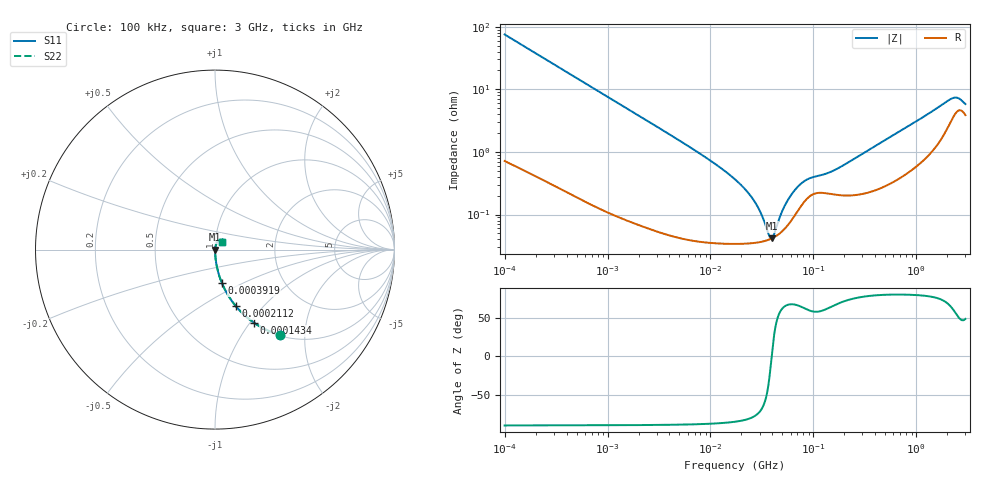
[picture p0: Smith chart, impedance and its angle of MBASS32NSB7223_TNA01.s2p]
! MBASS32NSB7223_TNA01  S-PARAMETER MODEL  ( Standard Model )
! Model Generated by TAIYO YUDEN Corporation (http://www.ty-top.com)
! Version 1.0
! TAIYO YUDEN Control No. 220601
! Copyright(c) 2013 TAIYO YUDEN CO.,LTD. All Rights Reserved.
! Product Description (link to TY-COMPAS)
! https://ds.yuden.co.jp/TYCOMPAS/or/detail?pn=MBASS32NSB7223KTNA01&u=M
! Products Name : Multilayer Ceramic Capacitors
! Characteristics :
!  Capacitance : 0.022 [uF] , Rated Voltage : 630 [V] , TCC : X7R
!  Case Size : 3.2 x 2.5 / 0.126 x 0.098 [mm/inch] , Thickness : 1.9 / 0.075 [mm/inch]
!  (Conditions: Temperature = 25 [degC] , DC Bias Voltage = 0 [V])
! External Node Assignments :
!  1  o---| |---o  2
! GND o---------o GND
! Frequency Range : 100kHz  -  3GHz  [ 401 STEP ]
# MHZ S RI R 50
! Freq[MHz].  S11 Real  S11 Imag  S21 Real  S21 Imag  S12 Real  S12 Imag  S22 Real  S22 Imag
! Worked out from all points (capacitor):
!   401 points, 100 kHz to 3 GHz, reference 50 ohm
!   read as one part in series: C = 21.2 nF near 105.3 kHz
!   lowest |Z| = 41.7 mohm at 39.51 MHz (marker M1)
!   series resonance near 39.35 MHz, so ESL is about 770 pH
!   S11 on the Smith chart (normalised r, x): 100 kHz: 1.01, -1.50; 143.4 kHz: 1.01, -1.05; 211.2 kHz: 1.01, -0.71; 391.9 kHz: 1.00, -0.39; 3 GHz: 1.08, +0.09
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0.1  0.3619 -0.4758  0.6381 0.4758  0.6381 0.4758  0.3619 -0.4758
0.14345  0.2183 -0.408  0.7817 0.408  0.7817 0.408  0.2183 -0.408
0.21115  0.116 -0.3147  0.884 0.3147  0.884 0.3147  0.116 -0.3147
0.391939  0.0381 -0.1856  0.9619 0.1856  0.9619 0.1856  0.0381 -0.1856
0.562235  0.0196 -0.1323  0.9804 0.1323  0.9804 0.1323  0.0196 -0.1323
3.161081  0.00111 -0.0241  0.9989 0.0241  0.9989 0.0241  0.00111 -0.0241
9.574722  0.000412 -0.00761  0.9996 0.00761  0.9996 0.00761  0.000412 -0.00761
17.7727  0.000352 -0.0035  0.9996 0.0035  0.9996 0.0035  0.000352 -0.0035
26.84345  0.000355 -0.00158  0.9996 0.00158  0.9996 0.00158  0.000355 -0.00158
31.3325  0.000368 -0.000932  0.9996 0.000932  0.9996 0.000932  0.000368 -0.000932
36.57227  0.000395 -0.0003  0.9996 0.0003  0.9996 0.0003  0.000395 -0.0003
39.51212  0.000417 1.74e-05  0.9996 -1.74e-05  0.9996 -1.74e-05  0.000417 1.74e-05
41.60216  0.000435 0.000231  0.9996 -0.000231  0.9996 -0.000231  0.000435 0.000231
51.12795  0.000565 0.00111  0.9994 -0.00111  0.9994 -0.00111  0.000565 0.00111
59.67813  0.000765 0.00181  0.9992 -0.00181  0.9992 -0.00181  0.000765 0.00181
75.25761  0.00134 0.00277  0.9987 -0.00277  0.9987 -0.00277  0.00134 0.00277
97.38194  0.00208 0.00332  0.9979 -0.00332  0.9979 -0.00332  0.00208 0.00332
167.3121  0.00208 0.00487  0.9979 -0.00487  0.9979 -0.00487  0.00208 0.00487
547.5153  0.00333 0.0167  0.9967 -0.0167  0.9967 -0.0167  0.00333 0.0167
2145.926  0.0324 0.0591  0.9676 -0.0591  0.9676 -0.0591  0.0324 0.0591
2504.792  0.0456 0.0532  0.9544 -0.0532  0.9544 -0.0532  0.0456 0.0532
3000  0.039 0.0402  0.961 -0.0402  0.961 -0.0402  0.039 0.0402
